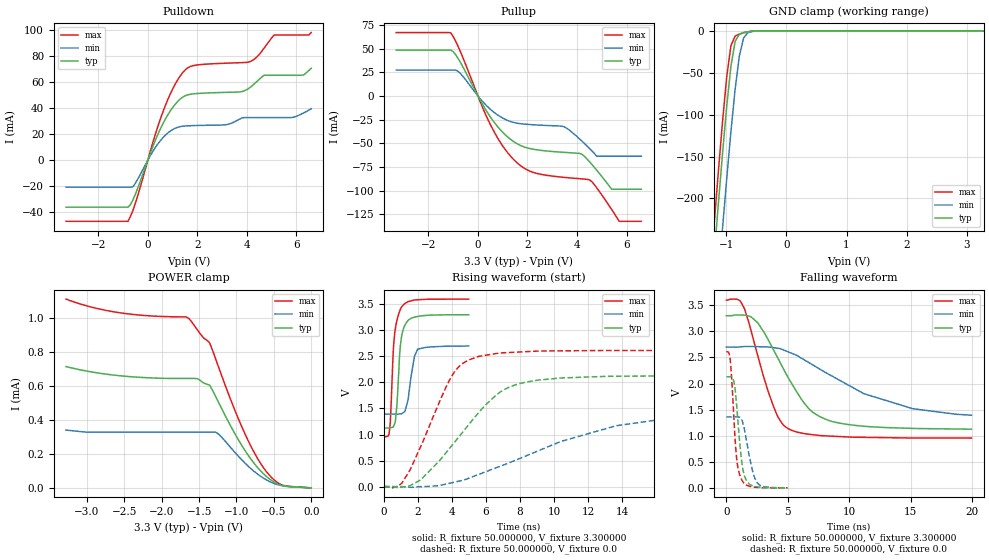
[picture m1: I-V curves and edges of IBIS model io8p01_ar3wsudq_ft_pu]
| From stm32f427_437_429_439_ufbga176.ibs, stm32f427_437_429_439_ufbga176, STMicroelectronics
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|   Model io8p01_ar3wsudq_ft_pu
[Model]  io8p01_ar3wsudq_ft_pu
Model_type I/O
Polarity   Non-Inverting
Enable   Active-Low
Vinl =   0.990000V
Vinh =   2.310000V
Vmeas =  1.650000V
Cref =   50.000000pF
Rref =   100.000000M
Vref =   0.0V
C_comp   3.843200pF   3.762100pF   3.937000pF
[Temperature Range]   25.000000   0.125000k   -40.000000
[Pullup Reference]   3.300000V   2.700000V   3.600000V
[Pulldown Reference]   0.0V   0.0V   0.0V
[POWER Clamp Reference]   3.300000V   2.700000V   3.600000V
[GND Clamp Reference]   0.0V   0.0V   0.0V
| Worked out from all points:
|   slope of the pulldown table from 0 to 0.495 V, typ, clamps not added: 20.9 ohm
|   slope of the pullup table from 0 to 0.495 V, typ, clamps not added: 22.6 ohm
|   GND clamp passes 1 mA (typ) near -0.62 V on its own axis
|   rising waveform, R_fixture 50.000000, V_fixture 3.300000: 20-80 % time 269ps typ, 352ps min, 281ps max; typ from 1.12 V to 3.3 V
|   rising waveform, R_fixture 50.000000, V_fixture 0.0: 20-80 % time 3.36ns typ, 6.9ns min, 2.12ns max; typ from 0.001 V to 2.13 V
|   falling waveform, R_fixture 50.000000, V_fixture 3.300000: 20-80 % time 3.22ns typ, 6.83ns min, 2.02ns max; typ from 3.3 V to 1.12 V
|   falling waveform, R_fixture 50.000000, V_fixture 0.0: 20-80 % time 505ps typ, 697ps min, 426ps max; typ from 2.13 V to 0.001 V
[Pulldown]
|Voltage   I(typ)   I(min)   I(max)
-3.3V     -36.18mA   -20.77mA   -47.07mA
-800mV    -36.18mA   -20.77mA   -47.07mA
-600mV    -30.5mA    -20.52mA   -38.69mA
700mV     31.4mA     19.11mA    41.71mA
1.2V      45.15mA    25.37mA    61.75mA
1.6V      50.35mA    26.5mA     71.06mA
3.1V      52.28mA    27.26mA    74.76mA
4.1V      55.65mA    32.89mA    75.79mA
4.7V      65.5mA     32.89mA    86.49mA
5.1V      65.5mA     32.89mA    96.55mA
6.3V      65.83mA    36.49mA    96.55mA
6.6V      70.88mA    39.7mA     98.4mA
[Pullup]
|Voltage   I(typ)   I(min)   I(max)
-3.3V     48.39mA    27.39mA    66.88mA
-1.1V     48.39mA    27.39mA    66.67mA
-700mV    35.09mA    23.45mA    46.27mA
500mV     -22.06mA   -14mA      -30.03mA
1.5V      -49.1mA    -28.3mA    -68.56mA
2.2V      -56.04mA   -30.32mA   -80.35mA
3.5V      -59.52mA   -32.72mA   -85.91mA
4.5V      -69.2mA    -55.26mA   -88.43mA
4.8V      -78.37mA   -63.6mA    -97mA
5.4V      -98.4mA    -63.6mA    -119.7mA
5.7V      -98.4mA    -63.6mA    -132.2mA
6.6V      -98.4mA    -63.6mA    -132.2mA
[GND_clamp]
|Voltage   I(typ)   I(min)   I(max)
-3.3V     -2.327A    -2.405A    -2.301A
-1.2V     -270.2mA   -361.4mA   -232.1mA
-1.13V    -207.3mA   -298.1mA   -169mA
-1.06V    -146.7mA   -236.2mA   -108.8mA
-990mV    -90.18mA   -176.4mA   -54.96mA
-920mV    -42.21mA   -120mA     -17.68mA
-850mV    -12.57mA   -69.47mA   -6.265mA
-780mV    -3.971mA   -30.01mA   -3.886mA
-710mV    -2.1mA     -8.615mA   -2.382mA
-640mV    -1.148mA   -2.283mA   -1.22mA
-570mV    -524uA     -821.5uA   -476.8uA
3.28V     0A         0A         0A
[POWER_clamp]
|Voltage   I(typ)   I(min)   I(max)
-3.28V    715.1uA    340.8uA    1.113mA
-2.6V     662.9uA    328.8uA    1.035mA
-1.64V    645uA      328.8uA    1mA
-1.52V    643.3uA    328.8uA    929.5uA
-1.36V    606.3uA    328.8uA    855.6uA
-1.24V    503.7uA    316.8uA    712.3uA
-960mV    272.5uA    179.4uA    391.9uA
-800mV    165.1uA    110.4uA    239.2uA
-640mV    83.2uA     57.57uA    119.3uA
-520mV    40.52uA    29.83uA    56.09uA
-400mV    15.54uA    13.29uA    18.7uA
0V        0A         0A         0A
[Ramp]
| variable   typ   min   max
dV/dt_r  1.27729/3.35985n   0.79875/6.90687n   1.56676/2.11512n
dV/dt_f  1.30152/3.21523n   0.73992/6.80411n   1.58714/2.02139n
R_load = 50.000000
[Rising Waveform]
R_fixture= 50.000000
V_fixture= 3.300000
V_fixture_min= 2.700000
V_fixture_max= 3.600000
|time   V(typ)   V(min)   V(max)
0s        1.125V     1.393V     955.6mV
360.4ps   1.128V     1.393V     1.187V
550.6ps   1.146V     1.393V     2.62V
660.7ps   1.238V     1.393V     3.006V
930.9ps   2.573V     1.395V     3.374V
1.031ns   2.867V     1.398V     3.443V
1.411ns   3.186V     1.658V     3.55V
1.782ns   3.251V     2.481V     3.582V
1.982ns   3.266V     2.637V     3.587V
4.985ns   3.3V       2.7V       3.599V
[Rising Waveform]
R_fixture= 50.000000
V_fixture= 0.0
V_fixture_min= 0.0
V_fixture_max= 0.0
|time   V(typ)   V(min)   V(max)
0s        1.445mV    1.247mV    1.817mV
1.041ns   -9.572mV   -268uV     61.62mV
2.162ns   130.6mV    -531.2uV   770.8mV
3.844ns   729.2mV    63.66mV    2.037V
4.364ns   938.5mV    102mV      2.288V
5.005ns   1.198V     164mV      2.434V
6.807ns   1.808V     388mV      2.565V
8.368ns   2.007V     592.6mV    2.591V
13.65ns   2.119V     1.168V     2.613V
19.94ns   2.129V     1.36V      2.612V
[Falling Waveform]
R_fixture= 50.000000
V_fixture= 3.300000
V_fixture_min= 2.700000
V_fixture_max= 3.600000
|time   V(typ)   V(min)   V(max)
0s        3.3V       2.7V       3.599V
920.9ps   3.315V     2.7V       3.612V
1.441ns   3.311V     2.71V      3.451V
2.563ns   3.163V     2.707V     2.53V
3.804ns   2.661V     2.689V     1.582V
5.045ns   2.109V     2.606V     1.134V
6.727ns   1.515V     2.4V       1.029V
8.609ns   1.273V     2.142V     991.7mV
15.14ns   1.141V     1.52V      957.7mV
19.94ns   1.125V     1.393V     955.6mV
[Falling Waveform]
R_fixture= 50.000000
V_fixture= 0.0
V_fixture_min= 0.0
V_fixture_max= 0.0
|time   V(typ)   V(min)   V(max)
0s        2.129V     1.36V      2.612V
300.3ps   2.131V     1.359V     2.49V
470.5ps   2.118V     1.359V     1.964V
620.6ps   2.031V     1.359V     1.317V
840.8ps   1.577V     1.361V     560.5mV
1.201ns   598.8mV    1.32V      181.1mV
1.592ns   163mV      968.4mV    60.49mV
2.152ns   38.89mV    305.8mV    15.61mV
2.472ns   20.61mV    113.3mV    10.55mV
4.985ns   1.445mV    1.247mV    1.817mV
